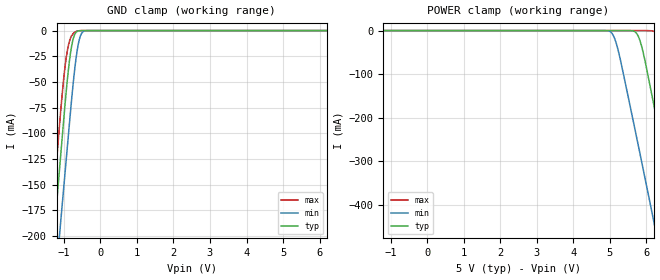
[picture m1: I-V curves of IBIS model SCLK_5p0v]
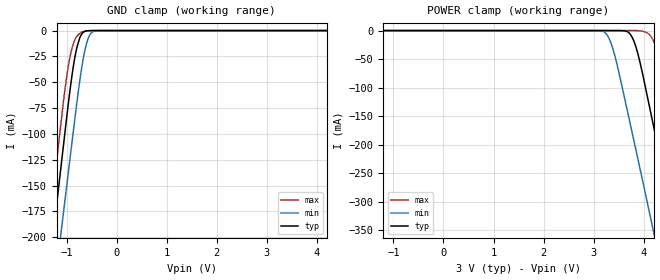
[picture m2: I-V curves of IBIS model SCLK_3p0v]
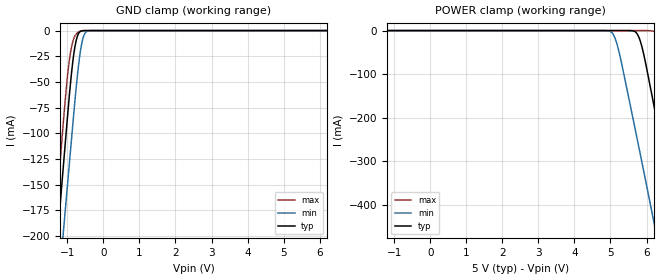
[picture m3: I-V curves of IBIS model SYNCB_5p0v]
|Texas Instruments Incorporated
| DAC084S085: 8-Bit Micro Power QUAD Digital-to-Analog Converter with
| Rail-to-Rail Output
| Marketing part#   Digital Voltage Range   Package-type   #pins
| DAC084S085CIMM   2.7 to 5.5 V   LLP   10
| DAC084S085CISD   2.7 to 5.5 V   MSOP   10
[IBIS Ver]   4.0
[File name]   dac084s085.ibs
[File Rev]   1.0
[Date]   01/19/2012
[Source]   Texas Instruments Incorporated.
   Analog-eLab, HPA
   12500 TI Blvd
   Dallas, TX -75243
   For Support e-mail: elab_ibis@list.ti.com
[Notes]   Revision History:
   1.0: 01/19/2012
   - Initial version of the model
   - Initial Model generated from simulations
   - Model not matched to measurements
   - Models with trailing _5p0v are generated based on 5.0V
   power supply.
   - Models with trailing _3p0v are generated based on 3.0V
   power supply.
   - C_comp although listed in numerical order of value are
   obtained from varying PVT conditions. For PVT conditions
   for each specific value refer the buffer description under
   respective [Model]. IBIS model user is responsible for using
   appropriate C_comp to simulate for Signal Integrity.
   - Combined pullup non-monotonic warnings for TXH,is based on
   SPICE simulations and accepted.
[Disclaimer]
  This model is designed as an aid for customers of Texas Instruments.
  TI and its licensors and suppliers make no warranties, either expressed
  or implied, with respect to this model, including the warranties of
  merchantability or fitness for a particular purpose.  The model is
  provided solely on an "as is" basis.  The entire risk as to its quality
  and performance is with the customer.
[Copyright] (C) Copyright 2012 Texas Instruments Incorporated.
   All rights reserved.
|   Device
[Component]   DAC084S085CIMM
[Manufacturer] TI
[Package]   | 10 pin LLP
| variable   typ   min   max
R_pkg   0.01   0.008   0.12
L_pkg   0.1nH   0.08nH   0.12nH
C_pkg   0.1pF   0.08pF   0.12pF
|-------------------------PIN------------------------------------------------
[Pin] signal_name  model_name  R_pin  L_pin C_pin
1   VA   POWER   NA   NA   NA
2   VOUTA   TERM   NA   NA   NA
3   VOUTB   TERM   NA   NA   NA
4   VOUTC   TERM   NA   NA   NA
5   VOUTD   TERM   NA   NA   NA
6   GND   GND   NA   NA   NA
7   VREFIN   TERM   NA   NA   NA
8   DIN   SCLK   NA   NA   NA
9   SYNCB   SYNCB   NA   NA   NA
10   SCLK   SCLK   NA   NA   NA
11   PAD   GND   NA   NA   NA
[Component]   DAC084S085CISD
[Manufacturer] TI
[Package]   | 10 pin MSOP
| variable   typ   min   max
R_pkg   0.01   0.008   0.12
L_pkg   0.1nH   0.08nH   0.12nH
C_pkg   0.1pF   0.08pF   0.12pF
|-------------------------PIN------------------------------------------------
[Pin] signal_name  model_name  R_pin  L_pin C_pin
1   VA   POWER   NA   NA   NA
2   VOUTA   TERM   NA   NA   NA
3   VOUTB   TERM   NA   NA   NA
4   VOUTC   TERM   NA   NA   NA
5   VOUTD   TERM   NA   NA   NA
6   GND   GND   NA   NA   NA
7   VREFIN   TERM   NA   NA   NA
8   DIN   SCLK   NA   NA   NA
9   SYNCB   SYNCB   NA   NA   NA
10   SCLK   SCLK   NA   NA   NA
11   PAD   GND   NA   NA   NA
[Model Selector] SCLK
SCLK_5p0v   model for 5.0v operation
SCLK_3p0v   model for 3.0v operation
[Model Selector] SYNCB
SYNCB_5p0v   model for 5.0v operation
SYNCB_3p0v   model for 3.0v operation
[Model Selector] TERM
TERM_5p0v   model for 5.0v operation
TERM_3p0v   model for 3.0v operation
|   Model
[Model] TERM_5p0v
Model_type Terminator
C_comp   1fF   1fF   1fF
| variable   typ   min   max
[Voltage Range]   5.0V   4.5V   5.5V
[POWER Clamp Reference]  3.3V   3.0V   3.6V
[GND Clamp Reference]   0.0V   0.0V   0.0V
|Operating Temperature
[Temperature Range]   27   85   -40
|   Model
[Model] TERM_3p0v
Model_type Terminator
C_comp   1fF   1fF   1fF
| variable   typ   min   max
[Voltage Range]   3.0V   2.7V   3.3V
[POWER Clamp Reference]  3.3V   3.0V   3.6V
[GND Clamp Reference]   0.0V   0.0V   0.0V
|Operating Temperature
[Temperature Range]   27   85   -40
| Models and submodels in the file (6): SCLK_5p0v (Input), SCLK_3p0v (Input), SYNCB_5p0v (Input), SYNCB_3p0v (Input), TERM_5p0v (Terminator), TERM_3p0v (Terminator)
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|   Model
[Model]   SCLK_5p0v
Model_type   Input
Vinl = 0.8
Vinh = 2.4
|   typ   min   max
C_comp   0.662pF   0.641pF   0.770pF
[Voltage Range]   5   4.5   5.5
[Temperature Range]   27   125   -40
[Power Clamp Reference]   5   4.5   5.5
[GND Clamp Reference]   0   0   0
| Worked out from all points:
|   GND clamp passes 1 mA (typ) near -0.64 V on its own axis
[GND Clamp]
|   Voltage   I(typ)   I(min)   I(max)
-5V       -1.813A    -1.827A    -1.812A
-1.355V   -235.3mA   -295.2mA   -195.6mA
-1.325V   -222.5mA   -282.9mA   -182.5mA
-1.235V   -184.3mA   -246.3mA   -143.1mA
-1.115V   -133.7mA   -197.8mA   -90.75mA
-995mV    -83.26mA   -149.6mA   -43.85mA
-905mV    -48.31mA   -113.7mA   -19.81mA
-785mV    -14.76mA   -66.35mA   -4.887mA
-635mV    -791uA     -19.45mA   -496.3uA
-515mV    -40.35uA   -2.742mA   -21.44uA
-365mV    -522.8nA   -51.88uA   0A
9.985V    0A         0A         0A
[POWER Clamp]
|   Voltage   I(typ)   I(min)   I(max)
-5V       0A         0A         0A
5.005V    0A         -2.188mA   0A
5.095V    0A         -11.61mA   0A
5.215V    0A         -41.65mA   0A
5.755V    -9.682mA   -254.4mA   0A
5.905V    -48.32mA   -315.6mA   -469.1nA
6.205V    -171.6mA   -439.3mA   -1.751mA
6.265V    -197mA     -464.2mA   -3.842mA
6.475V    -286.4mA   -551.6mA   -37.4mA
6.865V    -453.8mA   -714.9mA   -200mA
7.495V    -725.9mA   -979.8mA   -477.9mA
9.985V    -1.807A    -2.032A    -1.583A
|   Model
[Model]   SCLK_3p0v
Model_type   Input
Vinl = 0.6
Vinh = 2.1
|   typ   min   max
C_comp   0.662pF   0.641pF   0.770pF
[Voltage Range]   3   2.7   3.3
[Temperature Range]   27   125   -40
[Power Clamp Reference]   3   2.7   3.3
[GND Clamp Reference]   0   0   0
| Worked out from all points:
|   GND clamp passes 1 mA (typ) near -0.64 V on its own axis
[GND Clamp]
|   Voltage   I(typ)   I(min)   I(max)
-3V       -944.7mA   -981.9mA   -923.4mA
-1.515V   -303.5mA   -360.8mA   -266mA
-1.317V   -219.1mA   -279.6mA   -179mA
-1.299V   -211.5mA   -272.3mA   -171.1mA
-1.173V   -158.1mA   -221.2mA   -116mA
-1.065V   -112.6mA   -177.7mA   -69.97mA
-885mV    -41.41mA   -105.7mA   -16.13mA
-795mV    -16.74mA   -70.15mA   -5.511mA
-687mV    -2.697mA   -33.01mA   -1.325mA
-561mV    -129.5uA   -6.787mA   -80.95uA
-417mV    -2.66uA    -222.4uA   -711.5nA
5.991V    0A         0A         0A
[POWER Clamp]
|   Voltage   I(typ)   I(min)   I(max)
-3V       0A         0A         0A
3.201V    0A         -1.993mA   0A
3.399V    -1.563uA   -36.62mA   0A
3.741V    -7.748mA   -168.1mA   -1.778uA
3.867V    -35.57mA   -218.8mA   -94.98uA
4.065V    -112.6mA   -299.2mA   -3.844mA
4.191V    -165.7mA   -350.9mA   -17.18mA
4.335V    -226.8mA   -410.3mA   -58.22mA
4.659V    -365.2mA   -545mA     -197.4mA
4.803V    -427.1mA   -605.1mA   -260.7mA
5.163V    -582.3mA   -756mA     -419.5mA
5.991V    -940.8mA   -1.105A    -786.3mA
|   Model
[Model]   SYNCB_5p0v
Model_type   Input
Vinl = 0.8
Vinh = 2.4
|   typ   min   max
C_comp   0.660pF   0.639pF   0.767pF
[Voltage Range]   5   4.5   5.5
[Temperature Range]   27   125   -40
[Power Clamp Reference]   5   4.5   5.5
[GND Clamp Reference]   0   0   0
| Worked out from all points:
|   GND clamp passes 1 mA (typ) near -0.64 V on its own axis
[GND Clamp]
|   Voltage   I(typ)   I(min)   I(max)
-5V       -1.813A    -1.827A    -1.812A
-1.355V   -235.3mA   -295.2mA   -195.6mA
-1.325V   -222.5mA   -282.9mA   -182.5mA
-1.235V   -184.3mA   -246.3mA   -143.1mA
-1.115V   -133.7mA   -197.8mA   -90.75mA
-995mV    -83.26mA   -149.6mA   -43.85mA
-905mV    -48.31mA   -113.7mA   -19.81mA
-785mV    -14.76mA   -66.35mA   -4.887mA
-635mV    -791uA     -19.45mA   -496.3uA
-515mV    -40.35uA   -2.742mA   -21.44uA
-365mV    -522.7nA   -51.88uA   0A
9.985V    0A         0A         0A
[POWER Clamp]
|   Voltage   I(typ)   I(min)   I(max)
-5V       0A         0A         0A
5.005V    0A         -2.188mA   0A
5.095V    0A         -11.61mA   0A
5.215V    0A         -41.65mA   0A
5.755V    -9.682mA   -254.4mA   0A
5.905V    -48.32mA   -315.6mA   -469.1nA
6.205V    -171.6mA   -439.3mA   -1.751mA
6.265V    -197mA     -464.2mA   -3.842mA
6.475V    -286.4mA   -551.6mA   -37.4mA
6.865V    -453.8mA   -714.9mA   -200mA
7.495V    -725.9mA   -979.8mA   -477.9mA
9.985V    -1.807A    -2.032A    -1.583A
